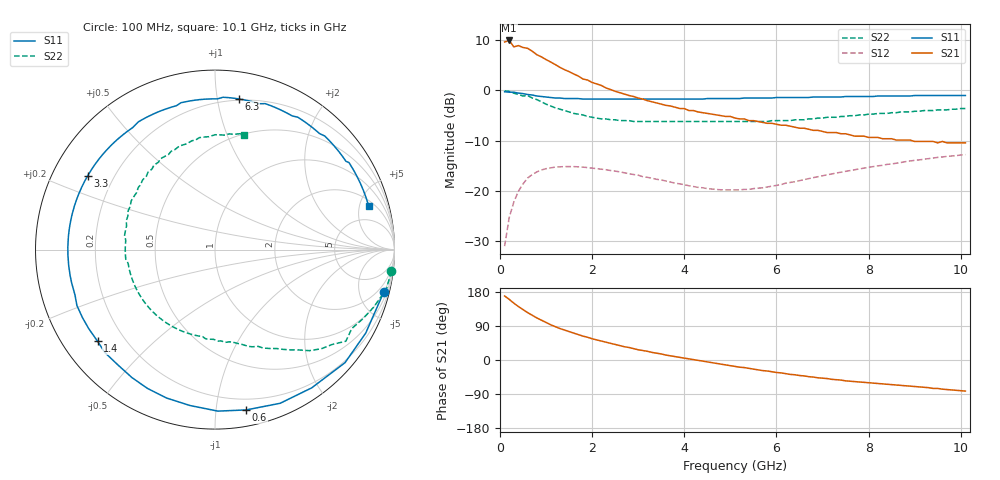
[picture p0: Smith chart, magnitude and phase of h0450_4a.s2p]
!HBFP-0450
!S and NOISE PARAMETERS at Vce=4V  Ic=1mA.  LAST UPDATED  09-04-98
# GHZ S MA R  50
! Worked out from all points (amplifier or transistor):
!   101 points, 100 MHz to 10.1 GHz, reference 50 ohm
!   highest |S21| = 10.0 dB at 200 MHz (marker M1)
!   |S21| within 3 dB of that: start of sweep to 835.8 MHz
!   unconditionally stable (mu >= 1): 3.295 GHz to end of sweep
!   at 1.7 GHz: K = 0.37, MSG = 9.0 dB, |S12| = -15.2 dB
!   at 5.1 GHz: K = 1.81, MAG = 2.0 dB, |S12| = -19.8 dB
!   at 10.1 GHz: K = 1.27, MAG = -1.9 dB, |S12| = -12.8 dB
!   lowest NFmin = 1.77 dB at 1.8 GHz
!   S11 on the Smith chart (normalised r, x): 100 MHz: 1.01, -8.02; 600 MHz: 0.12, -1.21; 1.4 GHz: 0.10, -0.34; 3.3 GHz: 0.11, +0.27; 6.3 GHz: 0.19, +1.15; 10.1 GHz: 2.56, +6.05
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0.1  0.97 -14.0  3.04 169.0  0.028 81.0  0.99 -7.0
0.2  0.96 -29.0  3.15 160.0  0.054 72.0  0.98 -13.0
0.3  0.96 -41.0  2.72 150.0  0.077 64.0  0.94 -20.0
0.4  0.94 -55.0  2.8 141.0  0.099 57.0  0.91 -25.0
0.6  0.91 -79.0  2.63 125.0  0.134 43.0  0.89 -35.0
0.7  0.9 -89.0  2.46 118.0  0.145 37.0  0.84 -39.0
0.8  0.88 -99.0  2.27 111.0  0.154 31.0  0.81 -43.0
1  0.86 -116.0  2.03 99.0  0.166 22.0  0.73 -50.0
1.2  0.84 -130.0  1.81 88.0  0.172 14.0  0.67 -56.0
1.4  0.83 -142.0  1.61 79.0  0.174 7.0  0.63 -61.0
1.8  0.82 -162.0  1.3 63.0  0.172 -4.0  0.57 -71.0
2.2  0.82 -178.0  1.12 50.0  0.164 -13.0  0.52 -81.0
2.5  0.82 172.0  0.98 41.0  0.157 -18.0  0.51 -88.0
3.3  0.82 150.0  0.77 20.0  0.133 -27.0  0.49 -108.0
3.5  0.82 145.0  0.73 16.0  0.128 -28.0  0.49 -113.0
4.5  0.83 121.0  0.59 -5.0  0.105 -28.0  0.49 -137.0
5.1  0.83 107.0  0.53 -17.0  0.102 -23.0  0.49 -152.0
6.3  0.85 81.0  0.44 -38.0  0.121 -17.0  0.5 174.0
6.8  0.86 71.0  0.4 -45.0  0.135 -18.0  0.52 159.0
8.5  0.88 41.0  0.33 -65.0  0.185 -33.0  0.6 114.0
9.2  0.89 30.0  0.31 -72.0  0.206 -42.0  0.63 98.0
10.1  0.89 16.0  0.3 -82.0  0.229 -56.0  0.66 76.0
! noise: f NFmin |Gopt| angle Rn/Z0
1.8  1.77  0.74  150  0.1
2  2  0.7  160  0.08
2.5  2.36  0.73  180  0.05
3.5  2.88  0.79  -149  0.26
4  3.2  0.81  -136  0.57
5  3.91  0.83  -111  1.79
5.5  3.9  0.88  -99  2.83
7  4.7  0.89  -67  6.91
8  5.19  0.9  -50  9.91
10  5.88  0.84  -18  12.41
